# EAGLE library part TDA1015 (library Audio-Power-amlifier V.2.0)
The TDA1015 is a monolithic integrated audio amplifier circuit in a 9-lead single in-line (SIL) plastic package. The device is especially designed for portable radio and recorder applications and delivers up to 4 W in a 4 W load impedance. The very low applicable supply voltage of 3,6 V permits 6 V applications.
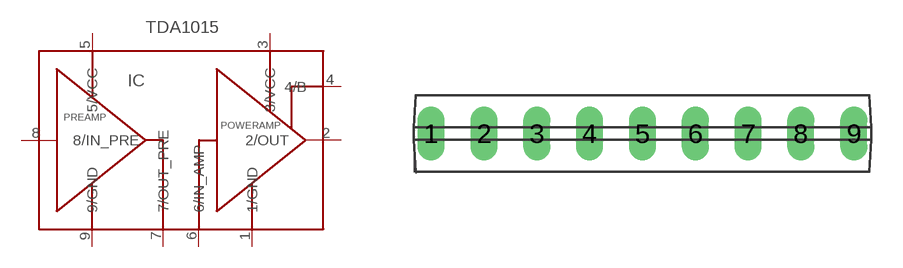
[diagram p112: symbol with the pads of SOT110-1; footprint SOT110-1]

Designator prefix IC

## TDA1015  [SOT110-1]
1  1/GND  pwr
2  2/OUT  out
3  3/VCC  pwr
4  4/B
5  5/VCC  pwr
6  6/IN_AMP  in
7  7/OUT_PRE  out
8  8/IN_PRE  in
9  9/GND  pwr

## Footprint SOT110-1 (pad centres in mm)
SIL9MPF: plastic single in-line medium power package with fin; 9 leads
drill 0.8 long: 1 -10.16,0; 2 -7.62,0; 3 -5.08,0; 4 -2.54,0; 5 0,0; 6 2.54,0; 7 5.08,0; 8 7.62,0; 9 10.16,0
